(* Logix 5000 AddOnInstructionDefinition export ACS_START_MOTION; software revision 20.01 *)

ADD_ON_INSTRUCTION ACS_START_MOTION   (* revision 2.0, vendor Tolomatic, Inc *)
VAR_IN_OUT
   DriveCMD : SINT; {required}   // ACS.O.CMD
END_VAR
VAR_INPUT
   PulseWidth : DINT := 200; {visible}   // Time to hold Start Motion bit High in Milliseconds. **This should be greater than the RPI of the drive
END_VAR
VAR_IN_OUT
   StartMotionTimer : TIMER; {required}   // Timer to hold Start Motion Bit High
   SMTimerEnable : BOOL; {required}   // Enable Line for Start Motion Timer
END_VAR

ROUTINE Logic   (* ladder *)
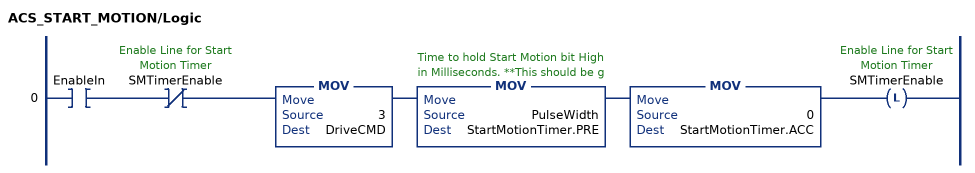
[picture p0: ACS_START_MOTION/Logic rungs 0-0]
   0: XIC(EnableIn)XIO(SMTimerEnable)MOV(3,DriveCMD)MOV(PulseWidth,StartMotionTimer.PRE)MOV(0,StartMotionTimer.ACC)OTL(SMTimerEnable);
END_ROUTINE
END_ADD_ON_INSTRUCTION
